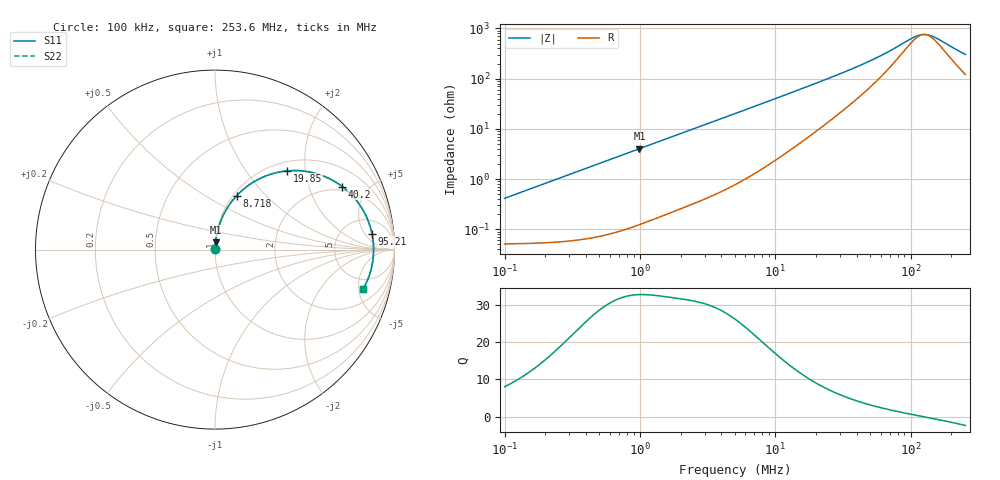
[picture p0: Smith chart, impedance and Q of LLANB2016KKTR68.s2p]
! LLANB2016KKTR68  S-PARAMETER MODEL  ( General Type )
! Model Generated by TAIYO YUDEN Corporation (http://www.ty-top.com)
! Version 1.0
! TAIYO YUDEN Control No. 120417NG38SB-FKC
! Copyright(c) 2012 TAIYO YUDEN CO.,LTD. All Rights Reserved.
! Product Description (link to TY-COMPAS)
! https://ds.yuden.co.jp/TYCOMPAS/or/detail?pn=LLANB2016KKTR68M&u=M
! Products Name : Inductors
! Characteristics :
!  Inductance : 0.68 uH , SRF(min) : -Hz , DC Resistance(max) : 0.065 Ohm
!  Rated Current : Saturation :2500 mA , Temp Rise : 2500 mA (40 degC)
!  Case Size : 2.0 x 1.6 / 0.079 x 0.063 [mm/inch] , Thickness : 1 / 0.039 [mm/inch]
!  (Conditions: Temperature = 25 degC , DC Bias Current/Voltage = 0A / 0V)
! External Node Assignments :
!  1  o---GGG---o  2
! GND o---------o GND
! Frequency Range : 0.1MHz  -  253.640152MHz  [ 402 STEP ]
# MHz S RI R 50
! Freq[MHz].  S11 Real  S11 Imag  S21 Real  S21 Imag  S12 Real  S12 Imag  S22 Real  S22 Imag
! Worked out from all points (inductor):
!   401 points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, 100 kHz to 253.6 MHz, reference 50 ohm
!   read as one part in series: L = 652 nH near 104 kHz
!   highest Q = 32.7 at 990.2 kHz (marker M1), where L = 647 nH
!   self-resonance near 126 MHz
!   S11 on the Smith chart (normalised r, x): 100 kHz: 1.00, +0.01; 8.718 MHz: 1.04, +0.70; 19.85 MHz: 1.18, +1.60; 40.2 MHz: 1.80, +3.37; 95.21 MHz: 10, +8; 253.6 MHz: 3.42, -5.56
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0.1  0.000526 0.00409  0.9995 -0.00409  0.9995 -0.00409  0.000526 0.00409
0.371712  0.000854 0.0152  0.9991 -0.0152  0.9991 -0.0152  0.000854 0.0152
0.990225  0.00284 0.0401  0.9972 -0.0401  0.9972 -0.0401  0.00284 0.0401
1.381698  0.00483 0.0556  0.9952 -0.0556  0.9952 -0.0556  0.00483 0.0556
2.797645  0.0159 0.11  0.9841 -0.11  0.9841 -0.11  0.0159 0.11
5.03627  0.0456 0.1903  0.9544 -0.1903  0.9544 -0.1903  0.0456 0.1903
8.717747  0.1207 0.3003  0.8793 -0.3003  0.8793 -0.3003  0.1207 0.3003
12.65041  0.2208 0.3803  0.7792 -0.3803  0.7792 -0.3803  0.2208 0.3803
18.72042  0.3768 0.4355  0.6232 -0.4355  0.6232 -0.4355  0.3768 0.4355
19.85396  0.4035 0.4387  0.5965 -0.4387  0.5965 -0.4387  0.4035 0.4387
27.70297  0.5581 0.4252  0.4419 -0.4252  0.4419 -0.4252  0.5581 0.4252
40.20007  0.7086 0.3515  0.2914 -0.3515  0.2914 -0.3515  0.7086 0.3515
52.8901  0.7889 0.2729  0.2111 -0.2729  0.2111 -0.2729  0.7889 0.2729
69.58603  0.842 0.1868  0.158 -0.1868  0.158 -0.1868  0.842 0.1868
95.21179  0.8748 0.0875  0.1252 -0.0875  0.1252 -0.0875  0.8748 0.0875
107.0913  0.8807 0.0507  0.1193 -0.0507  0.1193 -0.0507  0.8807 0.0507
115.8234  0.8829 0.0262  0.1171 -0.0262  0.1171 -0.0262  0.8829 0.0262
125.2675  0.8837 0.00176  0.1163 -0.00176  0.1163 -0.00176  0.8837 0.00176
135.4817  0.8831 -0.0227  0.1169 0.0227  0.1169 0.0227  0.8831 -0.0227
155.4012  0.8788 -0.0656  0.1212 0.0656  0.1212 0.0656  0.8788 -0.0656
216.8371  0.8493 -0.1708  0.1507 0.1708  0.1507 0.1708  0.8493 -0.1708
253.6402  0.8246 -0.2206  0.1754 0.2206  0.1754 0.2206  0.8246 -0.2206
